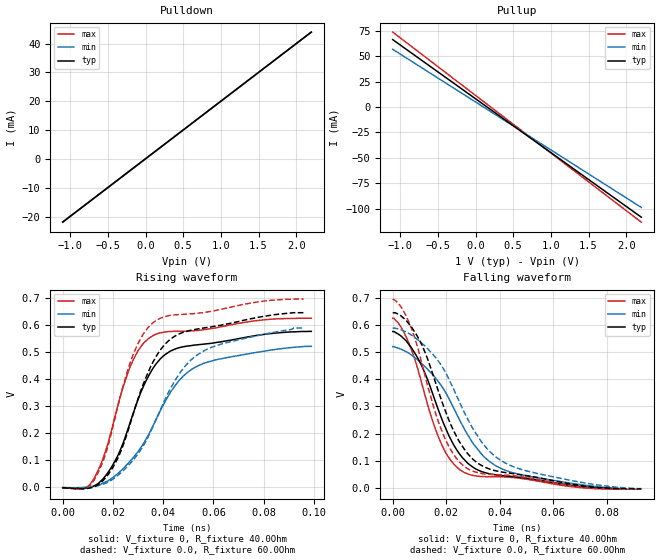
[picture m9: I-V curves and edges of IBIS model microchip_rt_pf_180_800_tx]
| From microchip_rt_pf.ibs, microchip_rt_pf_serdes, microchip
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[Model]   microchip_rt_pf_180_800_tx
Model_type   Output
Polarity   Non-Inverting
Enable   Active-High
Vmeas = 0.5
|   typ   min   max
C_comp   0.407p  0.407p  0.407p
[Voltage Range]   1.0  0.9  1.1
[Temperature Range]   27  27  27
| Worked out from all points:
|   slope of the pulldown table from 0 to 0.15 V, typ, clamps not added: 50.1 ohm
|   slope of the pullup table from 0 to 0.15 V, typ, clamps not added: 18.9 ohm
|   rising waveform, V_fixture 0, R_fixture 40.0Ohm: 20-80 % time 15.8ps typ, 21.2ps min, 13ps max; typ from -0.002 V to 0.576 V
|   rising waveform, V_fixture 0.0, R_fixture 60.0Ohm: 20-80 % time 16.7ps typ, 21.7ps min, 13.9ps max; typ from -0.003 V to 0.645 V
|   falling waveform, V_fixture 0, R_fixture 40.0Ohm: 20-80 % time 15.6ps typ, 20.6ps min, 12.9ps max; typ from 0.576 V to -0.003 V
|   falling waveform, V_fixture 0.0, R_fixture 60.0Ohm: 20-80 % time 16.6ps typ, 21.6ps min, 13.9ps max; typ from 0.645 V to -0.004 V
[Pullup]
|   X   TYP   MIN   MAX
-1.1V     66.22mA    56.71mA    73.61mA
1.01V     -45.41mA   -42.73mA   -45.89mA
1.089V    -49.57mA   -46.44mA   -50.34mA
2.2V      -108.3mA   -98.8mA    -113.3mA
[Pulldown]
|   X   TYP   MIN   MAX
-1.1V     -21.83mA   -21.87mA   -21.79mA
1.01V     20.27mA    20.25mA    20.28mA
1.089V    21.83mA    21.82mA    21.84mA
2.2V      44mA       44mA       44mA
[Ramp]
R_load = 50.0Ohm
|   typ   min   max
dV/dt_r   3.47E-1V/1.58E-2ns   3.14E-1V/2.12E-2ns   3.76E-1V/1.30E-2ns
dV/dt_f   3.47E-1V/1.56E-2ns   3.14E-1V/2.06E-2ns   3.77E-1V/1.29E-2ns
[Rising Waveform]
V_fixture   = 0
V_fixture_min = 0
V_fixture_max = 0
R_fixture   = 40.0Ohm
|   Time   V(typ)   V(min)   V(max)
0s        -2.5mV     -2mV       -2.5mV
8ps       -4.501mV   -2mV       -6.007mV
12ps      1.963mV    2.511mV    23.86mV
16ps      29.36mV    14.05mV    104.2mV
20ps      82.21mV    35.15mV    231.4mV
27ps      243mV      97.47mV    447.9mV
35ps      424.6mV    208.5mV    554.5mV
44ps      507.6mV    365.5mV    576mV
53ps      525.6mV    444.5mV    579mV
99ps      576mV      520.5mV    624.5mV
[Rising Waveform]
V_fixture   = 0.0
V_fixture_min = 0.0
V_fixture_max = 0.0
R_fixture   = 60.0Ohm
|   Time   V(typ)   V(min)   V(max)
0s        -3mV       -2.5mV     -3mV
11ps      -3.518mV   -480.9uV   7.436mV
18ps      44.65mV    17.75mV    150.4mV
23ps      128.5mV    51.19mV    337.1mV
27ps      238mV      88.71mV    463.4mV
32ps      378.8mV    151.1mV    565.1mV
36ps      463.3mV    224.6mV    608.3mV
46ps      565mV      412.8mV    637.9mV
55ps      586.7mV    497.6mV    644.4mV
96ps      645mV      588.5mV    695.5mV
[Falling Waveform]
V_fixture   = 0
V_fixture_min = 0
V_fixture_max = 0
R_fixture   = 40.0Ohm
|   Time   V(typ)   V(min)   V(max)
0s        576mV      520.5mV    624.5mV
5ps       542.1mV    501.7mV    556.7mV
10ps      466.6mV    466.1mV    416.5mV
14ps      373.6mV    427.1mV    275.3mV
18ps      263.3mV    379.3mV    166.7mV
21ps      192.9mV    329.9mV    111.8mV
25ps      125.2mV    251mV      67.86mV
33ps      61.1mV     127.2mV    42.36mV
41ps      45.55mV    69.67mV    40.86mV
85ps      -2.995mV   -2mV       -4mV
[Falling Waveform]
V_fixture   = 0.0
V_fixture_min = 0.0
V_fixture_max = 0.0
R_fixture   = 60.0Ohm
|   Time   V(typ)   V(min)   V(max)
0s        645mV      588.5mV    695.5mV
5ps       617.5mV    574.3mV    633.2mV
10ps      544.2mV    540.8mV    493.1mV
15ps      418.7mV    492.1mV    308.4mV
19ps      301.6mV    438.7mV    194.8mV
27ps      139.8mV    273.9mV    77.79mV
35ps      74.4mV     147.8mV    50.8mV
44ps      54.28mV    82.84mV    45.83mV
72ps      6.561mV    17.83mV    990.3uV
93ps      -3.5mV     -2.5mV     -4.5mV
[Algorithmic Model]
Executable Linux_gcc5.4_64   MPF300T-TX_LX64.so   MPF300T-TX-R180_800.ami
Executable Windows_cl18.00.40629_64 MPF300T-TX_WIN64.dll  MPF300T-TX-R180_800.ami
Executable Windows_cl18.00.40629_32 MPF300T-TX_WIN32.dll  MPF300T-TX-R180_800.ami
[End Algorithmic Model]
